FUNCTION_BLOCK FB_SFP_PPD_IO_LINK_CYCLIC_PROTOKOL_V1_0_0

   VAR_INPUT 
	  	  	
	  b_RELEASE_FUNKTION_BLOCK : BOOL; 
      b_00_FAST_STOP : BOOL;
      b_02_ACKNOLEDGE : BOOL;
      b_06_REPEAT_COMMAND_TOGGLE : BOOL;
      b_07_GRIP_DIREKTION : BOOL;
	  b_08_JOG_MODE_NEGATIVE : BOOL;
      b_09_JOG_MODE_POSITIVE : Bool;
      b_10_EXHAUST : BOOL;
      b_11_CALIBRATE : BOOL;
      b_16_MOVE_TO_ABSOLUTE_POSITION : BOOL;
      b_17_MOVE_TO_RELATIVE_POS : BOOL;
	  b_18_FULLY_CLOSE : BOOL;
	  b_19_FULLY_OPEN : BOOL;
	  b_20_GRIP_WORKPIECE : BOOL;
	  b_21_GRIP_WORKPIECE_AT_EXPECTED_POSITION : BOOL;
	  b_22_CLOSE_ALL_VALVES : BOOL;
	  
	  si_GAIN : SINT;
	  si_SPEED : SINT;
	  i_TARGET_ACCURANCY  : INT;
	  di_TARGET_POSITION : DINT;
	  
	  dw_IN_STATUS_DWORD_GRIPPER : DWORD;
      by_IN_WARNING_CODE : BYTE;
      by_IN_ERROR_CODE : BYTE;
      di_IN_ACTUAL_POSITION : DINT;
	  i_IN_ACTUAL_PRESSURE_DIFFERENCE : INT;
   END_VAR

   VAR_OUTPUT 
	  
      b_00_READY_FOR_OPPERATION : Bool;
      b_01_CONTOL_AUTHORITY_FIELDBUS : Bool;
      b_03_NOT_FEASIBLE : BOOL;
      b_04_SENSOR_CALIBRATED : BOOL;
      b_05_COMMAND_RECEIVED_TOGGLE : BOOL;
      b_06_WARNING : Bool;
      b_07_ERROR : Bool;
      b_08_ALL_VALVES_CLOSED : BOOL;
      b_09_EXHAUSTED : BOOL;
      b_16_POSITION_REACHED : BOOL;
      b_17_NO_WORKPIECE_DETECTED : BOOL;
      b_18_WORKPIECE_GRIPPED : BOOL;
      b_19_WRONG_WORKPIECE_DETECTED : BOOL;
      b_20_WORKPIECE_LOST : BOOL;


      by_WARNING_CODE : BYTE;
      by_ERROR_CODE : BYTE;
      di_ACTUAL_POSITION : DINT;
	  i_ACTUAL_PRESSURE_DIFFERENCE :INT;
	  
      dw_OUT_CONTROL_DW_GRIPPER : DWORD;
	  si_OUT_GAIN : SINT;
	  si_OUT_SPEED : SINT;
	  i_OUT_TARGET_ACCURANCY  : INT;
	  di_OUT_TARGET_POSITION : DINT;
	  
   END_VAR
   
   
   VAR_TEMP 
	  b_Temp_OUT_0 : BOOL;
	  b_Temp_OUT_1 : BOOL;
	  b_Temp_OUT_2 : BOOL;
	  b_Temp_OUT_3 : BOOL;
	  b_Temp_OUT_4 : BOOL;
	  b_Temp_OUT_5 : BOOL;
	  b_Temp_OUT_6 : BOOL;	   
	  b_Temp_OUT_7 : BOOL;
	  b_Temp_OUT_8 : BOOL;
	  b_Temp_OUT_9 : BOOL;	  
	  b_Temp_OUT_10 : BOOL;
	  b_Temp_OUT_11 : BOOL;
	  b_Temp_OUT_12 : BOOL;
  	  b_Temp_OUT_13 : BOOL;
  	  b_Temp_OUT_14 : BOOL;
      b_Temp_OUT_15 : BOOL;
      b_Temp_OUT_16 : BOOL;
      b_Temp_OUT_17 : BOOL;	  
	  b_Temp_OUT_18 : BOOL;
	  b_Temp_OUT_19 : BOOL;
	  b_Temp_OUT_20 : BOOL;
	  b_Temp_OUT_21 : BOOL;
	  b_Temp_OUT_22 : BOOL;
	  b_Temp_OUT_23 : BOOL;
	  b_Temp_OUT_24 : BOOL;
	  b_Temp_OUT_25 : BOOL;
	  b_Temp_OUT_26 : BOOL;
	  b_Temp_OUT_27 : BOOL;
	  b_Temp_OUT_28 : BOOL;
	  b_Temp_OUT_29 : BOOL;
	  b_Temp_OUT_30 : BOOL;
      b_Temp_OUT_31 : BOOL;
	  
	  b_Temp_IN_1 : BOOL;
	  b_Temp_in_2 : BOOL;
	  b_Temp_in_3 : BOOL;
	  b_Temp_in_4 : BOOL;
	  b_Temp_in_5 : BOOL;
	  b_Temp_in_6 : BOOL;
	  b_Temp_in_7 : BOOL;
	  b_Temp_in_8 : BOOL;
	  b_Temp_in_9 : BOOL;
	  b_Temp_in_10 : BOOL;
	  b_Temp_in_11 : BOOL;
	  b_Temp_in_12 : BOOL;
	  b_Temp_in_13 : BOOL;
	  b_Temp_in_14 : BOOL;
	  b_Temp_in_15 : BOOL;
	  b_Temp_in_16 : BOOL;
	  b_Temp_in_17 : BOOL;
	  b_Temp_in_18 : BOOL;
	  b_Temp_in_19 : BOOL;
	  b_Temp_in_20 : BOOL;
	  b_Temp_in_21 : BOOL;
	  b_Temp_in_22 : BOOL;
	  b_Temp_in_23 : BOOL;
	  b_Temp_in_24 : BOOL;
	  b_Temp_in_25 : BOOL;
	  b_Temp_in_26 : BOOL;
	  b_Temp_in_27 : BOOL;
	  b_Temp_in_28 : BOOL;
	  b_Temp_in_29 : BOOL;
	  b_Temp_in_30 : BOOL;
	  b_Temp_in_31 : BOOL;
	  	  
   END_VAR



	(*
	FUNCTION_BLOCK FB_SFP_Cyclic_Protokol
	TITLE = 'FB_SFP_EGU_EGK_IO_Link_Cyclic_Protocol'
	VERSION : '1.0.0'
	AUTHOR  : 'SCHUNK'
	NAME    : 'FB_Zyklische_Kommunikation_SFP_Beckhoff TwinCAT 3'
	FAMILY  : 'SCHUNK'
	Projekt Nr.:
	=============================================================================
	 Schunk GmbH&Co.KG
	 (c)Copyright (2023) All Rights Reserved
	-----------------------------------------------------------------------------
	 Library:       Schunk
	 Tested with:   TWINCAT 3 Build 4024.47
	 Engineering:   TWINCAT 3 Build 4024.47
	 Restrictions:  XXX(OB types, etc.)
	 Requirements:  (hardware, technological package, memory needed, etc.)
	 Functionality: The Funktion Block communicates Cyclic with the Gripper to read and Wright Data
	  
	*************************************************************************
	Historie
	
	####################
	1.0.0
	Release Funktion Block
	
	
	*************************************************************************)
	
// MANUAL ENGLISH 
    
    // Statement section REGION
    
    (*************************************************************************    
    The function block is TO read AND transfer cyclic parameters that are changed FOR specific functions in the device
    can be used TO make The application process safer OR faster.
    
    Input parameters:
    ------------------
    b_RELEASE_FUNCTION_BLOCK            : Release FOR processing the block
    
    b_00_FAST_STOP                      : immediate shutdown of The process currently running in the gripper and shutdown of the motor phases
    b_02_ACKNOLEDGE                     : As long as the PPD is in error state and if an acknowledge was triggered, the PPD shall check if there are still any error causes.
                                          If there are no error causes any more, the state shall change to operational.
                                          Operational readiness is not established (again).
                                          If there are still any error causes, the status shall remain in error state and transmit the latest error code.
    b_06_REPEAT_COMMAND_TOGGLE          : The command that is still pending can, if it is a repeatable command, be repeated without loss OF Time for each positive and negative change of this bit
    b_07_GRIP_DIRECTION                 : determines The gripping direction. FALSE = external gripping (the workpiece is gripped from the outside) / True = internal gripping (the workpiece is gripped from the inside).
    
    b_08_JOG_MODE_NEGATIVE              : The gripper shall execute a movement with a fix velocity in the control bit corresponding direction.
                                          The value of the used fix velocity shall be 1 mm/s.
                                          Negative means a movement in the direction of decreasing position values. Function is also possible without "Calibration".
    b_09_JOG_MODE_POSITIVE              : The gripper shall execute a movement with a fix velocity in the control bit corresponding direction.
                                          The value of the used fix velocity shall be 1 mm/s.
                                          Positive means a movement in the direction of increasing position values. Function is also possible without "Calibration".
    b_10_EXHAUST                        : As soon as this function has been triggered the PPD shall open all valves to exhaust the air of both chambers.
                                          To trigger this function the PPD shall be in operation or error status.
    b_11_CALIBRATE                      : The calibrate function creates a routine in the PPD that determines the minimum and maximum position of the connected pneumatic product, 
                                          provided a measuring system is available. The routine runs automatically.
      
    b_16_MOVE_TO_ABSOLUTE_POSITION      : When executing the command, the PPD tries to move to the specified position "Tag Position".
                                          In order to be able to execute this function, further parameters must be transferred: target accuracy, speed, gain.
    b_17_MOVE_TO_RELATIVE_POSITION      : When the command is executed, the PPD attempts to move to the specified, calculated position.
                                          In order to be able to execute this function, further parameters must be transferred: target position, target accuracy, speed, gain.
    b_18_FULLY_CLOSE                    : With this function, the PPD executes a movement to the minimum possible position.
    b_18_FULLY_OPEN                     : With this function, the PPD executes a movement to the maximum possible position.
    b_20_GRIP_WORKPIECE                 : The gripper shall grip workpieces at a nonspecific position.
                                          To execute this function the following parameter values shall be transmitted.
                                                - target pressure difference
                                                - speed
                                                - grip direction (control bit)
    b_21_GRIP_WORKPIECE_AT_EXPECTED_POSITION : The gripper should grip workpieces at a specific position.
                                               To execute this function, the following parameter values must be transferred.
                                                     - target position
                                                     - target pressure difference
                                                     - speed
    b_22_CLOSE_ALL_VALVES               : As soon as this function has been triggered the PPD shall close all valves.
    
    si_GAIN                             : If a function needs a gain value to execute, the IO-Link master must transfer this value in the cyclic gain parameter.
                                          The gain value ranges from 1 to 10
    si_SPEED                            : If a function needs a speed value to execute, the IO-Link-Master shall transmit this value in the cyclic parameter speed.
                                          Valid values shall be 1 to 10.
    i_TARGET_ACCURANCY                  : The parameter must represent a value in micrometers [µm].
                                          Valid values are between 500 µm and 15,000 µm.
    di_TARGET_POSITION                  : Valid values shall be -5.000.000 µm to 5.000.000 µm.
    i_TARGET_PRESSURE_DIFFERENCE        : The target pressure difference shall represent the mathematical absolute value of the pressure difference between the two compression chambers.
                                          Valid values shall be 2000 mbar to 8.000 mbar.
  
    HW_ADRESS_INPUT                     : Indicates the input hardware address of the gripper from which the data is to be fetched
    HW_ADRESS_OUTPUT                    : Indicates the Output hardware address of the gripper to which the data is to be written
    #################
    
    
    Output parameters:
    ------------------
    
    b_00_READY_FOR_OPERATION            : indicates that the gripper is ready FOR operation
    b_01_CONTOL_AUTHORITY_FIELDBUS      : indicates whether the fieldbus has control authority over the gripper
    b_03_NOT_FEASIBLE                   : Indicates that the last issued command cannot be executed.
                                            Possible causes are:
                                            - a new command was sent although the command that is still active has NOT yet been processed.
                                            - 2 OR more control commands simultaneously active in the control word
                                            - Parameter data FOR position, speed OR force are outside the permissible limits.
    
    b_04_SENSOR_CALIBRATED              : indicates that the "Calibrate" command was executed correctly and the sensor is calibrated
    b_05_COMMAND_RECEIVED_TOGGLE        : indicates that a command was sent to The gripper via the bus. the command does not have TO be processed or started at the time it is displayed.
    b_06_WARNING                        : signals a warning in the gripper, e.g. temperature warning
    b_07_ERROR                          : signals a fault in the gripper, e.g. rapid stop
    b_08_ALL_VALVES_CLOSED              : indicates that all Valves are closed 
    b_09_EXHAUSTED                      : indicates that the EXHAUST funktion is completed successfully
    
    b_16_POSITION_REACHED               : signals that the relative or absolute position has been approached
    b_17_NO_WORKPIECE_DETECTED          : indicates that no workpiece was detected
    b_18_WORKPIECE_GRIPPED              : signals that a workpiece has been gripped
    b_19_WRONG_WORKPIECE_DETECTED       : signals that a wrong workpiece was detected
    b_20_WORKPIECE_LOST                 : signals that the gripped workpiece was lost
    
    by_WARNING_CODE                     : Output of the gripper's warning code
    by_ERROR_CODE                       : Output of the error code of the gripper
    
    di_ACTUAL_POSITION                  : the current position OF The gripper is returned here
    i_ACTUAL_PRESSURE_DIFFERENCE        : As long as a workpiece is being gripped, the IO-Link master should be able to evaluate the actual signed pressure difference value by reading out the cyclic parameter actual pressure difference.
                                          The value is shown in millibar [mbar].
    
    *************************************************************************)
    
// MANUAL GERMAN
    
(*************************************************************************
    Der Baustein soll Zyklische Parameter einlesen und übertragen, welche für bestimmte Funktionen im Gerät geändert 
    werden können um den Applikationsprozess sicherer oder schneller zu machen.
    
    Eingangsparameter:
    ------------------
    
    b_RELEASE_FUNCTION_BLOCK            : Freigabe zur Bearbeitung des Bausteins (True = Freigabe zur Bearbeitung)
    
    b_00_FAST_STOP                      : Sobald diese Funktion ausgelöst wird, wird jede Bewegung abgebrochen und der PPD in den Fehlerzustand versetzt.
    b_02_ACKNOLEDGE                     : Solange sich das PPD im Fehlerzustand befindet und eine Bestätigung ausgelöst wurde, prüft das PPD, ob noch Fehlerursachen vorliegen.
                                          Liegen keine Fehlerursachen mehr vor, wechselt der Zustand in „Operational“.
                                          Die Betriebsbereitschaft ist nicht (wieder) hergestellt.
                                          Liegen weiterhin Fehlerursachen vor, bleibt der Status im Fehlerzustand und übermittelt den aktuellsten Fehlercode.
    b_06_REPEAT_COMMAND_TOGGLE          : Das Noch anstehende Kommando kann, sofern es ein wiederholbares Kommando ist, ohne Zeitverlust bei jedem positiven und negativen Wechsel dieses Bits wiederholt werden 
    b_07_GRIP_DIRECTION                 : legt die Greifrichtung fest. FALSE = Ausengreifen (Das Werkstück wird von außen gegriffen) / True = Innengreifen (Das Werkstück wird von innen gegriffen). 
    
    b_08_JOG_MODE_NEGATIVE              : Der Greifer soll eine Bewegung mit fester Geschwindigkeit in die dem Steuerbit entsprechende Richtung ausführen.
                                          Der Wert der verwendeten Fixgeschwindigkeit muss 1 mm/s betragen.
                                          Negativ bedeutet eine Bewegung in Richtung abnehmender Positionswerte. Funktion ist auch ohne „Kalibrierung“ möglich.
    b_09_JOG_MODE_POSITIVE              : Der Greifer soll eine Bewegung mit fester Geschwindigkeit in die dem Steuerbit entsprechende Richtung ausführen.
                                          Der Wert der verwendeten Fixgeschwindigkeit muss 1 mm/s betragen.
                                          Positiv bedeutet eine Bewegung in Richtung steigender Positionswerte. Funktion ist auch ohne „Kalibrierung“ möglich.
    b_10_EXHAUST                        : Sobald diese Funktion ausgelöst wurde, öffnet die PPD alle Ventile, um die Luft aus beiden Kammern abzulassen.
                                          Um diese Funktion auszulösen, muss sich die PPD im Betriebs- oder Fehlerstatus befinden.
    b_11_CALIBRATE                      : Die Funktion Kalibrieren stertet in der PPD eine Rutiene welche die minimale und maximale Position der angeschlossenen Pneumatischen produktes ermittelt, 
                                          sofern ein Messsystem vorhanden ist. Die Routine läuft selbständig ab. 
    
    b_16_MOVE_TO_ABSOLUTE_POSITION      : Beim ausführen des Befehls versucht die PPD aud die vorgegebene Position "Taget Position" zu fahren.
                                          Um diese Funktion ausführen zu können, müssen weitere Parameter übertragen werden: target accurancy, Speed, Gain
    b_17_MOVE_TO_RELATIVE_POSITION      : Beim ausführen des Befehls versucht die PPD auf die vorgegebene errechnete Position zu fahren.
                                          Um diese Funktion ausführen zu können, müssen weitere Parameter übertragen werden: target possition, target accurancy, Speed, Gain.
    b_18_FULLY_CLOSE                    : Bei dieser Funktion führt die PPD eine Bewegung auf die minimal mögliche Position aus. 
    b_19_FULLY_OPEN                     : Bei dieser Funktion führt die PPD eine Bewegung auf die maximal mögliche Position aus. 
    b_20_GRIP_WORKPIECE                 : Der Greifer soll Werkstücke an einer unbestimmten Position greifen.
                                          Zur Ausführung dieser Funktion müssen folgende Parameterwerte übertragen werden.
                                                - target pressure difference
                                                - speed
                                                - grip direction (control bit)
                                          
    b_21_GRIP_WORKPIECE_AT_EXPECTED_POSITION    : Der Greifer soll Werkstücke an einer bestimmten Position greifen.
                                                  Zur Ausführung dieser Funktion müssen folgende Parameterwerte übertragen werden.
                                                        - target position
                                                        - target pressure difference
                                                        - speed
    b_22_CLOSE_ALL_VALVES               : Sobald diese Funktion ausgelöst wurde, soll das PPD alle Ventile schließen.
    
    
    si_GAIN                             : Wenn eine Funktion zur Ausführung einen Verstärkungswert benötigt, muss der IO-Link-Master diesen Wert im zyklischen Parameter Verstärkung übertragen.
                                          Der Wert der Verstärkung bewegt sich zwischen 1 und 10
    si_SPEED                            : Benötigt eine Funktion zur Ausführung einen Geschwindigkeitswert, muss der IO-Link-Master diesen Wert im zyklischen Parameter Geschwindigkeit übertragen.
                                          Gültige Werte liegen zwischen 1 und 10.
    i_TARGET_ACCURANCY                  : Der Parameter muss einen Wert in Mikrometern [µm] darstellen.
                                          Gültige Werte liegen zwischen 500 µm und 15.000 µm.
    di_TARGET_POSITION                  : Gültige Werte liegen zwischen -5.000.000 µm und 5.000.000 µm.
    i_TARGET_PRESSURE_DIFFERENCE        : Die Zieldruckdifferenz soll den mathematischen Absolutwert der Druckdifferenz zwischen den beiden Kompressionskammern darstellen.
                                          Gültige Werte liegen zwischen 2000 mbar und 8.000 mbar.
    

    ##################    
    
    
    Ausgangsparameter:
    ------------------
    
    b_00_READY_FOR_OPPERATION           : zeigt die Betriebsbereitschaft des Greifers an
    b_01_CONTOL_AUTHORITY_FIELDBUS      : zeigt an, ob der Feldbus die Steuerhoheit über den Greifer hat
    b_03_NOT_FEASIBLE                   : Zeigt an, das der zuletzt abgesetzte Befehl nicht ausgeführt werden kann.
                                            Mögliche Ursachen sind:
                                            - ein neuer Befehl wurde abgesetzt, obwohl der noch aktive Befehl noch nicht abgearbeitet wurde.
                                            - 2 oder mehr Steuerbefehle gleichzeitig aktiv im Steuerwort
                                            - Parameterdaten von Position, Geschwindigkeit oder Kraft liegen auserhalb der Zulässigen grenzen. 
                                
    b_04_SENSOR_CALIBRATED              : Zeigt an das der Befehl "Calibrate" korrekt ausgeführt wurde und der Sensor Kalibriert ist
    b_05_COMMAND_RECEIVED_TOGGLE        : Zeigt an das ein Befehl über den Bus an den Greufer gesendet wurde. Zum Zeitpunkt der Anzeige muß der Befehl noch nicht abgearbeitet oder gestartet sein.
    b_06_WARNING                        : signalisiert eine Warnung im Greifer, z.B. Temperaturwarnung
    b_07_ERROR                          : signalisiert eine Störung im Greifer, z.B. Schnellstop
    b_08_ALL_VALVES_CLOSED              : zeigt an, dass alle Ventile geschlossen sind
    b_09_EXHAUSTED                      : zeigt an, dass die EXHAUST-Funktion erfolgreich abgeschlossen wurde
    
    b_16_POSITION_REACHED               : signalisiert, dass die relative oder absolute Position angefahren wurde
    b_17_NO_WORKPIECE_DETECTED          : signalisiert, dass kein Werkstück erkannt wurde
    b_18_WORKPIECE_GRIPPED              : signalisiert, dass ein Werkstück gegriffen wurde
    b_19_WRONG_WORKPIECE_DETECTED       : signalisiert, das ein falsches Werkstück erkannt wurde
    b_20_WORKPIECE_LOST                 : signalisiert, dass das gegriffene Werkstück verloren ging
    
    by_WARNING_CODE                     : Ausgabe des Warnungscodes des Greifers
    by_ERROR_CODE                       : Ausgabe des Störungscodes des Greifers
    di_ACTUAL_POSITION                  : hier wird die aktuelle Possition des Greifers zurückgegeben
    i_ACTUAL_PRESSURE_DIFFERENCE        : Solange ein Werkstück gegriffen wird, soll der IO-Link-Master in der Lage sein, den tatsächlichen vorzeichenbehafteten Druckdifferenzwert durch Auslesen des zyklischen Parameters Ist-Druckdifferenz auszuwerten.
                                          Der Wert wird in millibar [mbar] dargestellt.
    
	*************************************************************************) 
	    
	// Release FB
	    // Statement section REGION
	    		
	    IF  
				b_RELEASE_FUNKTION_BLOCK = TRUE
	    THEN
	       
			b_00_READY_FOR_OPPERATION 			:= DW_IN_STATUS_DWORD_GRIPPER.0;
			b_01_CONTOL_AUTHORITY_FIELDBUS 		:= DW_IN_STATUS_DWORD_GRIPPER.1;
			b_Temp_OUT_2						:= DW_IN_STATUS_DWORD_GRIPPER.2;
			b_03_NOT_FEASIBLE 					:= DW_IN_STATUS_DWORD_GRIPPER.3;
			b_04_SENSOR_CALIBRATED				:= DW_IN_STATUS_DWORD_GRIPPER.4;
			b_05_COMMAND_RECEIVED_TOGGLE 		:= DW_IN_STATUS_DWORD_GRIPPER.5;
			b_06_WARNING 						:= DW_IN_STATUS_DWORD_GRIPPER.6;
			b_07_ERROR 							:= DW_IN_STATUS_DWORD_GRIPPER.7;
			b_08_ALL_VALVES_CLOSED				:= DW_IN_STATUS_DWORD_GRIPPER.8;
			b_09_EXHAUSTED			 			:= DW_IN_STATUS_DWORD_GRIPPER.9;
			b_Temp_OUT_10	 					:= DW_IN_STATUS_DWORD_GRIPPER.10;
			b_Temp_OUT_11						:= DW_IN_STATUS_DWORD_GRIPPER.11;
			b_Temp_OUT_12						:= DW_IN_STATUS_DWORD_GRIPPER.12;
			b_Temp_OUT_13						:= DW_IN_STATUS_DWORD_GRIPPER.13;
			b_Temp_OUT_14						:= DW_IN_STATUS_DWORD_GRIPPER.14;
			b_Temp_OUT_15 						:= DW_IN_STATUS_DWORD_GRIPPER.15; 
			b_16_POSITION_REACHED 				:= DW_IN_STATUS_DWORD_GRIPPER.16;
			b_17_NO_WORKPIECE_DETECTED			:= DW_IN_STATUS_DWORD_GRIPPER.17;
			b_18_WORKPIECE_GRIPPED				:= DW_IN_STATUS_DWORD_GRIPPER.18;
			b_19_WRONG_WORKPIECE_DETECTED		:= DW_IN_STATUS_DWORD_GRIPPER.19;
			b_20_WORKPIECE_LOST					:= DW_IN_STATUS_DWORD_GRIPPER.20;
			b_Temp_OUT_21 						:= DW_IN_STATUS_DWORD_GRIPPER.21;
			b_Temp_OUT_22 						:= DW_IN_STATUS_DWORD_GRIPPER.22;
			b_Temp_OUT_23 						:= DW_IN_STATUS_DWORD_GRIPPER.23;
			b_Temp_OUT_24 						:= DW_IN_STATUS_DWORD_GRIPPER.24; 
			b_Temp_OUT_25 						:= DW_IN_STATUS_DWORD_GRIPPER.25; 
			b_Temp_OUT_26 						:= DW_IN_STATUS_DWORD_GRIPPER.26; 
			b_Temp_OUT_27 						:= DW_IN_STATUS_DWORD_GRIPPER.27; 
			b_Temp_OUT_28 						:= DW_IN_STATUS_DWORD_GRIPPER.28; 
			b_Temp_OUT_29 						:= DW_IN_STATUS_DWORD_GRIPPER.29; 
			b_Temp_OUT_30 						:= DW_IN_STATUS_DWORD_GRIPPER.30; 
			b_Temp_OUT_31						:= DW_IN_STATUS_DWORD_GRIPPER.31; 
			
			di_ACTUAL_POSITION 					:= di_IN_ACTUAL_POSITION;
			by_WARNING_CODE 					:= by_IN_WARNING_CODE;
			by_ERROR_CODE						:= by_IN_ERROR_CODE;
			di_ACTUAL_POSITION					:= di_IN_ACTUAL_POSITION;
			i_ACTUAL_PRESSURE_DIFFERENCE		:= i_IN_ACTUAL_PRESSURE_DIFFERENCE;
 
			
			//*************************************************************************
			dw_OUT_CONTROL_DW_GRIPPER.0 := b_00_FAST_STOP;
			dw_OUT_CONTROL_DW_GRIPPER.1 := FALSE;
			dw_OUT_CONTROL_DW_GRIPPER.2 := b_02_ACKNOLEDGE;
			dw_OUT_CONTROL_DW_GRIPPER.3 := FALSE;
			dw_OUT_CONTROL_DW_GRIPPER.4 := FALSE;
			dw_OUT_CONTROL_DW_GRIPPER.5 := FALSE;
			dw_OUT_CONTROL_DW_GRIPPER.6 := b_06_REPEAT_COMMAND_TOGGLE;
			dw_OUT_CONTROL_DW_GRIPPER.7 := b_07_GRIP_DIREKTION;
			dw_OUT_CONTROL_DW_GRIPPER.8 := b_08_JOG_MODE_NEGATIVE;
			dw_OUT_CONTROL_DW_GRIPPER.9 := b_09_JOG_MODE_POSITIVE;
			dw_OUT_CONTROL_DW_GRIPPER.10 := b_10_EXHAUST;
			dw_OUT_CONTROL_DW_GRIPPER.11 := b_11_CALIBRATE;
			dw_OUT_CONTROL_DW_GRIPPER.12 := FALSE;
			dw_OUT_CONTROL_DW_GRIPPER.13 := FALSE;
			dw_OUT_CONTROL_DW_GRIPPER.14 := FALSE;
			dw_OUT_CONTROL_DW_GRIPPER.15 := FALSE;
			dw_OUT_CONTROL_DW_GRIPPER.16 := b_16_MOVE_TO_ABSOLUTE_POSITION;
			dw_OUT_CONTROL_DW_GRIPPER.17 := b_17_MOVE_TO_RELATIVE_POS;
			dw_OUT_CONTROL_DW_GRIPPER.18 := b_18_FULLY_CLOSE;
			dw_OUT_CONTROL_DW_GRIPPER.19 := b_19_FULLY_OPEN;
			dw_OUT_CONTROL_DW_GRIPPER.20 := b_20_GRIP_WORKPIECE;
			dw_OUT_CONTROL_DW_GRIPPER.21 := b_21_GRIP_WORKPIECE_AT_EXPECTED_POSITION;
			dw_OUT_CONTROL_DW_GRIPPER.22 := b_22_CLOSE_ALL_VALVES;
			dw_OUT_CONTROL_DW_GRIPPER.23 := FALSE;
			dw_OUT_CONTROL_DW_GRIPPER.24 := FALSE;
			dw_OUT_CONTROL_DW_GRIPPER.25 := FALSE;
			dw_OUT_CONTROL_DW_GRIPPER.26 := FALSE;
			dw_OUT_CONTROL_DW_GRIPPER.27 := FALSE;
			dw_OUT_CONTROL_DW_GRIPPER.28 := FALSE;
			dw_OUT_CONTROL_DW_GRIPPER.29 := FALSE;
			dw_OUT_CONTROL_DW_GRIPPER.30 := FALSE;
			dw_OUT_CONTROL_DW_GRIPPER.31 := FALSE;

			si_OUT_GAIN := si_GAIN;
			si_OUT_SPEED:= si_SPEED;
			i_OUT_TARGET_ACCURANCY:= i_TARGET_ACCURANCY;
			di_OUT_TARGET_POSITION:= di_TARGET_POSITION;
			
	    END_IF;

END_FUNCTION_BLOCK
